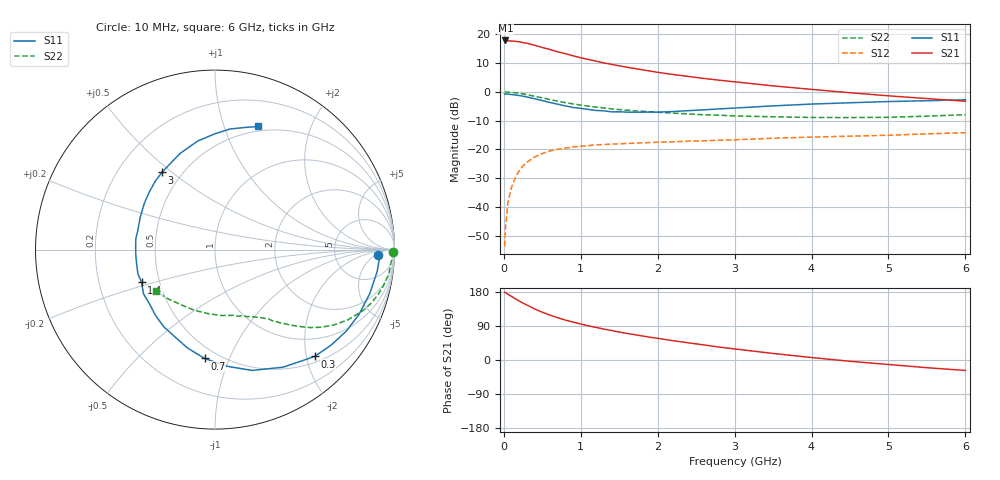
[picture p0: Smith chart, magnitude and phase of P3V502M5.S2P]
! SIEMENS Small Signal Semiconductors
! BFP181
! Si NPN RF Bipolar Junction Transistor in SOT143
! VCE = 0.5 V  IC = 2.5 mA
! Common Emitter S-Parameters:  March  1996
# GHz  S  MA  R  50
!  f  S11  S21  S12  S22
! GHz  MAG  ANG  MAG  ANG  MAG  ANG  MAG  ANG
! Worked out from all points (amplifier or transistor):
!   36 points, 10 MHz to 6 GHz, reference 50 ohm
!   highest |S21| = 17.8 dB at 20 MHz (marker M1)
!   |S21| within 3 dB of that: start of sweep to 581.8 MHz
!   unconditionally stable (mu >= 1): 1.777 GHz to end of sweep
!   at 250 MHz: K = 0.18, MSG = 21.4 dB, |S12| = -25.7 dB
!   at 1.4 GHz: K = 0.84, MSG = 13.8 dB, |S12| = -18.1 dB
!   at 6 GHz: K = 1.35, MAG = 1.9 dB, |S12| = -14.2 dB
!   S11 on the Smith chart (normalised r, x): 10 MHz: 19, -6; 300 MHz: 0.61, -2.16; 700 MHz: 0.42, -0.81; 1.4 GHz: 0.40, -0.18; 3 GHz: 0.39, +0.46; 6 GHz: 0.45, +1.30
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0.01  0.9104 -1.8  7.72 179.0  0.0021 86.2  0.9895 -0.7
0.02  0.9169 -3.4  7.769 178.1  0.0042 90.5  0.9907 -1.6
0.05  0.9116 -7.8  7.727 173.9  0.0114 86.8  0.9838 -4.1
0.1  0.8961 -16.0  7.572 167.8  0.0221 79.1  0.9775 -8.0
0.15  0.8801 -24.2  7.509 161.5  0.0326 75.4  0.9611 -11.9
0.25  0.8383 -39.2  7.123 150.1  0.052 66.8  0.9184 -19.1
0.3  0.8141 -47.0  6.947 145.1  0.0599 63.0  0.8931 -22.3
0.4  0.7573 -59.9  6.412 134.8  0.0739 56.0  0.8371 -27.9
0.5  0.704 -73.0  5.855 126.1  0.085 49.8  0.784 -32.4
0.6  0.6523 -84.4  5.424 118.3  0.0942 45.1  0.7338 -36.1
0.7  0.609 -95.5  4.933 111.6  0.1004 40.6  0.6875 -39.2
0.8  0.5693 -105.6  4.58 105.3  0.1055 37.3  0.6492 -41.5
0.9  0.5351 -114.7  4.213 100.1  0.1102 34.3  0.6158 -43.6
1.1  0.4942 -132.1  3.641 90.0  0.1168 29.8  0.5632 -47.0
1.4  0.448 -155.9  2.988 77.8  0.1238 24.9  0.5065 -51.3
1.8  0.4425 177.8  2.406 63.4  0.1302 21.4  0.4592 -55.8
2.2  0.4542 156.3  1.995 50.9  0.1358 18.6  0.4254 -61.4
3  0.5223 124.6  1.489 29.2  0.1471 14.5  0.3801 -74.5
3.5  0.5695 110.1  1.267 17.3  0.1564 12.6  0.3687 -84.8
4.5  0.6451 90.1  0.963 -3.4  0.17 6.9  0.3571 -108.8
5.5  0.6998 76.4  0.763 -20.3  0.1866 3.4  0.3778 -133.0
6  0.726 70.9  0.686 -27.6  0.1952 0.6  0.4009 -144.4
